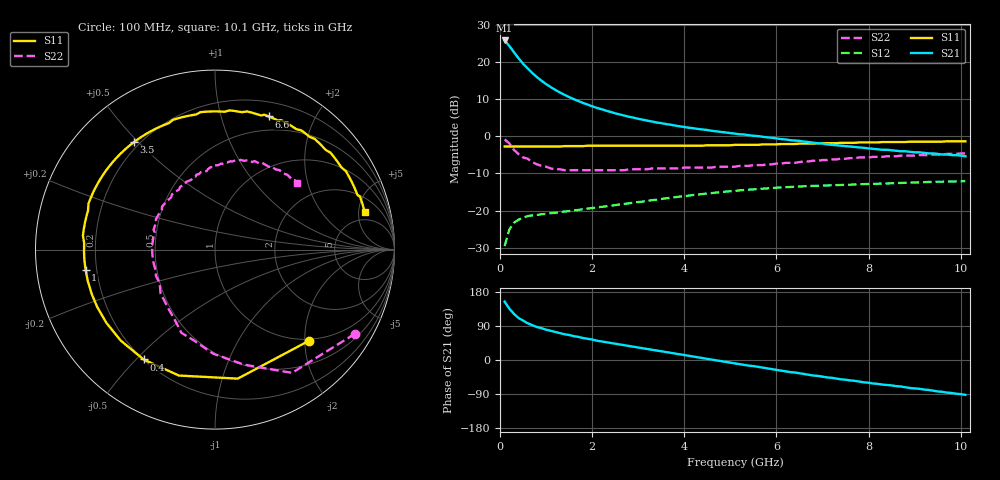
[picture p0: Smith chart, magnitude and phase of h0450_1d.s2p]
!HBFP-0450
!S and NOISE PARAMETERS at Vce=1V  Ic=10mA.  LAST UPDATED  09-04-98
# GHZ S MA R  50
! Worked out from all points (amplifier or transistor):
!   101 points, 100 MHz to 10.1 GHz, reference 50 ohm
!   highest |S21| = 25.9 dB at 100 MHz (marker M1)
!   |S21| within 3 dB of that: start of sweep to 293.1 MHz
!   unconditionally stable (mu >= 1): 2.61 GHz to end of sweep
!   at 1.7 GHz: K = 0.78, MSG = 14.7 dB, |S12| = -19.8 dB
!   at 5.1 GHz: K = 1.15, MAG = 5.4 dB, |S12| = -14.7 dB
!   at 10.1 GHz: K = 1.12, MAG = 1.3 dB, |S12| = -12.1 dB
!   lowest NFmin = 1.15 dB at 1.8 GHz
!   S11 on the Smith chart (normalised r, x): 100 MHz: 0.97, -2.10; 400 MHz: 0.20, -0.53; 1 GHz: 0.16, -0.08; 3.5 GHz: 0.18, +0.49; 6.6 GHz: 0.35, +1.43; 10.1 GHz: 3.68, +5.89
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0.1  0.73 -44.0  19.74 154.0  0.033 68.0  0.91 -31.0
0.2  0.73 -80.0  16.74 136.0  0.055 51.0  0.81 -58.0
0.3  0.73 -106.0  13.79 122.0  0.068 42.0  0.66 -76.0
0.4  0.73 -123.0  11.4 111.0  0.075 35.0  0.58 -91.0
0.5  0.73 -136.0  9.58 104.0  0.08 30.0  0.52 -103.0
0.6  0.73 -146.0  8.28 97.0  0.084 26.0  0.5 -112.0
0.7  0.73 -154.0  7.18 92.0  0.086 24.0  0.45 -120.0
0.8  0.73 -160.0  6.33 87.0  0.087 23.0  0.42 -128.0
0.9  0.73 -166.0  5.64 84.0  0.089 22.0  0.4 -135.0
1  0.73 -171.0  5.09 80.0  0.09 21.0  0.39 -141.0
1.2  0.73 -179.0  4.25 74.0  0.093 20.0  0.36 -151.0
1.4  0.74 174.0  3.64 68.0  0.097 20.0  0.35 -160.0
1.8  0.74 163.0  2.83 58.0  0.104 19.0  0.35 -174.0
2.1  0.75 155.0  2.43 51.0  0.11 18.0  0.35 178.0
2.5  0.75 146.0  2.05 43.0  0.118 17.0  0.35 168.0
3.5  0.75 127.0  1.51 23.0  0.143 11.0  0.37 150.0
4.3  0.75 112.0  1.26 7.0  0.164 4.0  0.38 136.0
5.1  0.77 96.0  1.09 -9.0  0.184 -5.0  0.39 121.0
6.6  0.8 68.0  0.85 -37.0  0.212 -25.0  0.46 93.0
6.8  0.8 64.0  0.82 -41.0  0.215 -27.0  0.47 90.0
8.5  0.84 38.0  0.65 -67.0  0.233 -48.0  0.54 65.0
10.1  0.86 14.0  0.54 -92.0  0.248 -70.0  0.59 39.0
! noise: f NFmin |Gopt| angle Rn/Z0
1.8  1.15  0.5  -179  0.04
2  1.22  0.52  -174  0.04
2.5  1.33  0.55  -159  0.06
3.5  1.64  0.63  -137  0.16
4  1.81  0.64  -124  0.28
5  2.11  0.69  -103  0.6
5.5  2.32  0.72  -92  0.86
7  2.73  0.76  -62  1.96
8  3.04  0.8  -46  2.87
10  3.59  0.81  -15  4.67
